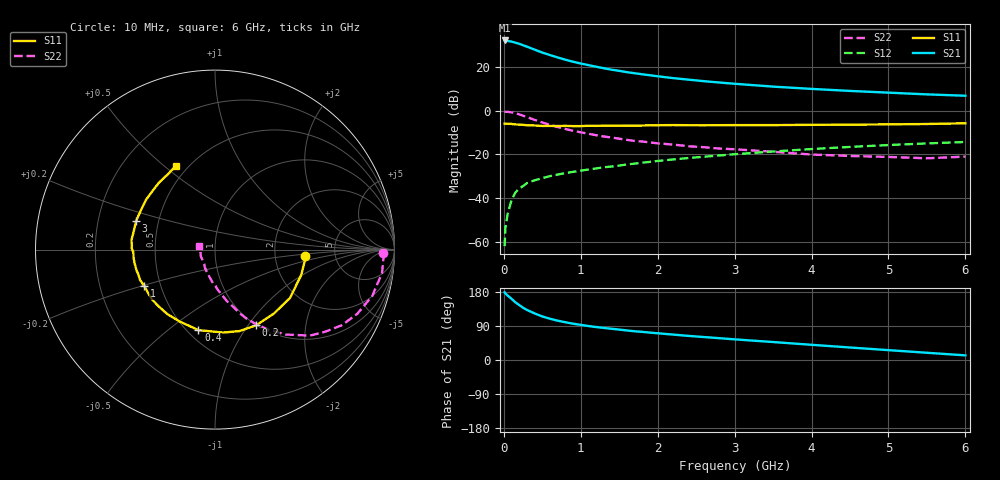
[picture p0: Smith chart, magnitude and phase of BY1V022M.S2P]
! SIEMENS Small Signal Semiconductors
! BFY420
! Si NPN RF SIEGET Grounded Emitter Transistor in MICRO-X
! VCE = 1 V  IC = 22 mA
! Common Emitter S-Parameters:  October  1996
# GHz  S  MA  R  50
!  f  S11  S21  S12  S22
! GHz  MAG  ANG  MAG  ANG  MAG  ANG  MAG  ANG
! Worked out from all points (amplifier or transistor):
!   36 points, 10 MHz to 6 GHz, reference 50 ohm
!   highest |S21| = 32.1 dB at 10 MHz (marker M1)
!   |S21| within 3 dB of that: start of sweep to 312 MHz
!   unconditionally stable (mu >= 1): start of sweep to 11.87 MHz; 1.654 GHz to end of sweep
!   at 250 MHz: K = 0.33, MSG = 32.2 dB, |S12| = -34.5 dB
!   at 1.4 GHz: K = 0.95, MSG = 22.1 dB, |S12| = -25.5 dB
!   at 6 GHz: K = 1.09, MAG = 8.7 dB, |S12| = -14.3 dB
!   S11 on the Smith chart (normalised r, x): 10 MHz: 3.00, -0.27; 200 MHz: 1.00, -1.09; 400 MHz: 0.57, -0.64; 1 GHz: 0.41, -0.21; 3 GHz: 0.37, +0.15; 6 GHz: 0.43, +0.55
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0.01  0.503 -3.9  40.17 178.8  0.0008 99.4  0.9378 -1.0
0.02  0.5043 -7.2  40.14 175.5  0.0021 96.0  0.9399 -2.7
0.05  0.5006 -16.6  38.95 170.0  0.0044 81.6  0.9397 -8.0
0.1  0.4972 -32.9  37.85 161.5  0.0091 80.9  0.9134 -16.4
0.15  0.4844 -47.4  35.77 152.1  0.0134 71.9  0.8702 -24.2
0.2  0.48 -61.4  33.71 145.1  0.0167 67.6  0.8227 -30.8
0.25  0.474 -73.3  31.27 137.9  0.0189 63.3  0.7648 -36.8
0.3  0.4645 -84.4  28.97 132.1  0.0221 62.2  0.7145 -42.1
0.4  0.458 -101.6  24.81 122.9  0.0256 58.0  0.6161 -50.2
0.5  0.4464 -116.1  21.22 114.9  0.0287 56.4  0.5366 -56.3
0.6  0.4468 -126.6  18.59 108.8  0.0319 55.2  0.4735 -61.2
0.7  0.4457 -135.0  16.43 103.7  0.0347 54.5  0.4229 -65.4
0.8  0.4477 -142.0  14.59 99.6  0.0374 53.2  0.3809 -68.8
1  0.4432 -152.6  11.93 92.7  0.0425 54.4  0.3201 -73.8
1.1  0.4507 -158.0  10.97 89.6  0.0451 54.6  0.2963 -76.8
1.6  0.456 -174.2  7.575 77.9  0.0587 54.5  0.215 -87.5
2.2  0.4688 173.4  5.541 67.1  0.0767 53.1  0.1677 -98.0
3  0.4676 159.8  4.112 54.5  0.101 48.5  0.1311 -110.5
3.5  0.4675 151.6  3.541 47.4  0.1164 44.9  0.115 -119.3
4.5  0.4772 137.0  2.823 33.0  0.1483 36.2  0.0921 -136.9
5.5  0.4955 121.9  2.353 19.1  0.1783 26.3  0.0815 -173.1
6  0.5144 115.1  2.191 12.2  0.1925 21.2  0.0891 167.9
